PROGRAM IL
VAR
	RANGE_PG_PS1:RANGEJD;
	RANGE_PG_PS2:RANGEJD;
	RANGE_PG_PS3:RANGEJD;
	RANGE_PG_PS4:RANGEJD;
	RANGE_PG_PS5:RANGEJD;
	RANGE_PG_PS6:RANGEJD;
	RANGE_PG_PS7:RANGEJD;
	RANGE_PG_PS8:RANGEJD;
	RANGE_PG_PS9:RANGEJD;
	
	RANGE_MFC1:RANGEJD;
	RANGE_MFC2:RANGEJD;
	RANGE_MFC3:RANGEJD;
	RANGE_MFC4:RANGEJD;
	RANGE_MFC5:RANGEJD;
	RANGE_MFC6:RANGEJD;
	RANGE_MFC7:RANGEJD;
	RANGE_MFC8:RANGEJD;
	RANGE_MFC9:RANGEJD;
	
	RANGE_CHAMBER_HEATER1:RANGEJD;
	RANGE_CHAMBER_HEATER2:RANGEJD;
	RANGE_CHAMBER_HEATER3:RANGEJD;
	
	RANGE_LID_HEATER:RANGEJD;
	
	RANGE_STAGE_EDGE_HEATER:RANGEJD;
	RANGE_STAGE_CENTER_HEATER:RANGEJD;
	
	//INTERLOCK	
	TON_PrepareTransfer:TON;	
	TON_TransferWafer:TON;	
	TON_OpenGasValve:TON;	
	TON_CloseGasValve:TON;	
	TON_OpenCloseSlitValve:TON;
	
	ALWAYS_TRUE:BOOL:=TRUE;
END_VAR
VAR // added by the converter: edge detectors and wires of the graphical bodies
    _w1, _w2, _w3, _w4, _w5, _w6 : BOOL;
END_VAR

VALVE();
Temp();
SYS();
SPLC();
ACT_HEATER();
ACT_MFC();
ACT_MFC();

//TMP Pressure OUT OF RANGE
	IF GV.PMConfig.TurboN2Pressure	<=	GV.TurboN2PurgePressure
		THEN
		PM.INFO.Alarm.TurboN2PurgePressureOutOfRange:=TRUE;
		ELSE
		PM.INFO.Alarm.TurboN2PurgePressureOutOfRange:=FALSE;	
	END_IF
	
//PrepareTransfer TIMEOUT
	TON_PrepareTransfer(IN:= GV_IL.STATUS_PrepareTransfer, PT:=INT_TO_TIME(GV.PMConfig.PrepareTransferTimeout)*1000 , Q=> , ET=> );	
	IF TON_PrepareTransfer.Q
		THEN
		PM.INFO.Alarm.PrepareTransferTimerout:=TRUE;
		ELSE
		PM.INFO.Alarm.PrepareTransferTimerout:=FALSE;
	END_IF
	
//TransferWafer TIMEOUT
	TON_TransferWafer(IN:=GV_IL.STATUS_TransferWafer , PT:= INT_TO_TIME(GV.PMConfig.TransferWaferTimeout)*1000, Q=> , ET=> );
	IF TON_TransferWafer.Q
		THEN
		PM.INFO.Alarm.TransferWaferTimeout:=TRUE;
		ELSE
		PM.INFO.Alarm.TransferWaferTimeout:=FALSE;	
	END_IF
	
//OpenGasValve TIMEOUT
	TON_OpenGasValve(IN:=GV_IL.STATUS_OpenGasValve , PT:= INT_TO_TIME(GV.PMConfig.OpenGasValveTimeout)*1000, Q=> , ET=> );
	IF TON_OpenGasValve.Q
		THEN
		PM.INFO.Alarm.OpenGasValveTimeout:=TRUE;
		ELSE 
		PM.INFO.Alarm.OpenGasValveTimeout:=FALSE;
	END_IF
	
//CloseGasValve TIMEOUT
	TON_CloseGasValve(IN:=GV_IL.STATUS_CloseGasValve , PT:= INT_TO_TIME(GV.PMConfig.CloseGasValveTimeout)*1000, Q=> , ET=> );
	IF TON_CloseGasValve.Q
		THEN
		PM.INFO.Alarm.CloseGasValveTimeout:=TRUE;
		ELSE
		PM.INFO.Alarm.CloseGasValveTimeout:=FALSE;
	END_IF
	
//OpenCloseSlitValve TIMEOUT
	TON_OpenCloseSlitValve(IN:=GV_IL.STATUS_OpenCloseSlitValve , PT:= INT_TO_TIME(GV.PMConfig.OpenCloseSlitValveTimeout)*1000, Q=> , ET=> );
	IF TON_OpenCloseSlitValve.Q
		THEN
		PM.INFO.Alarm.OpenCloseSlitValveTimeout:=TRUE;
		ELSE
		PM.INFO.Alarm.OpenCloseSlitValveTimeout:=FALSE;	
	END_IF
	
	
//PRESSURE ALARM
	//PM.INFO.Alarm.PRESSURE:=
	
//ALARM OR WARNING OCCUR
	GV.ALARM_OCC:=NOT (
				 	//PM.INFO.Alarm.PRESSURE
					PM.INFO.Alarm.MFC1	
				AND PM.INFO.Alarm.MFC2	
				AND	PM.INFO.Alarm.MFC3
				AND PM.INFO.Alarm.MFC4	
				AND PM.INFO.Alarm.MFC5	
				AND PM.INFO.Alarm.MFC6
				AND PM.INFO.Alarm.MFC7	
				AND PM.INFO.Alarm.MFC8	
				AND PM.INFO.Alarm.MFC9
				AND PM.INFO.Alarm.WALL_TEMP	
				AND PM.INFO.Alarm.LID_TEMP	
				AND PM.INFO.Alarm.STAGE_EDGE_TEMP	
				AND PM.INFO.Alarm.STAGE_CENTER_TEMP
				AND PM.INFO.Alarm.Gas1FlowPressureOutOfRange
				AND PM.INFO.Alarm.Gas2FlowPressureOutOfRange
				AND PM.INFO.Alarm.Gas3FlowPressureOutOfRange
				//AND PM.INFO.Alarm.Gas4FlowPressureOutOfRange
				AND PM.INFO.Alarm.Gas5FlowPressureOutOfRange
				AND PM.INFO.Alarm.Gas6FlowPressureOutOfRange
				//AND PM.INFO.Alarm.TurboN2PurgePressureOutOfRange
				//AND PM.INFO.Alarm.PrepareTransferTimerout
				//AND PM.INFO.Alarm.TransferWaferTimeout
				//AND PM.INFO.Alarm.OpenGasValveTimeout
				//AND PM.INFO.Alarm.CloseGasValveTimeout
				//AND PM.INFO.Alarm.OpenCloseSlitValveTimeout
				//AND PM.INFO.Alarm.ATMCheckTimeout
				//AND PM.INFO.Alarm.DRY_PUMP
				//AND PM.INFO.Alarm.PENDULUM_VALVE
				//AND PM.INFO.Alarm.TURBO_PUMP
				AND PM.INFO.Alarm.CHILLER1
				AND PM.INFO.Alarm.CHILLER2
				AND (PM.INFO.Alarm.TOLERANCE_PRESSURE				
				AND PM.INFO.Alarm.TOLERANCE_MFC1
				AND PM.INFO.Alarm.TOLERANCE_MFC2
				AND PM.INFO.Alarm.TOLERANCE_MFC3
				AND PM.INFO.Alarm.TOLERANCE_MFC4
				AND PM.INFO.Alarm.TOLERANCE_MFC5
				AND PM.INFO.Alarm.TOLERANCE_MFC6
				AND PM.INFO.Alarm.TOLERANCE_MFC7
				AND PM.INFO.Alarm.TOLERANCE_MFC8
				AND PM.INFO.Alarm.TOLERANCE_MFC9
				AND PM.INFO.Alarm.TOLERANCE_WALL_TEMP
				AND PM.INFO.Alarm.TOLERANCE_LID_TEMP
				AND PM.INFO.Alarm.TOLERANCE_STAGE_EDGE_TEMP
				AND PM.INFO.Alarm.TOLERANCE_STAGE_CENTER_TEMP)
				);

	GV.WARNING_OCC:=NOT (
					//PM.INFO.Warning.PRESSURE					
					PM.INFO.Warning.MFC1
				AND PM.INFO.Warning.MFC2
				AND PM.INFO.Warning.MFC3
				AND PM.INFO.Warning.MFC4
				AND PM.INFO.Warning.MFC5
				AND PM.INFO.Warning.MFC6
				AND PM.INFO.Warning.MFC7
				AND PM.INFO.Warning.MFC8
				AND PM.INFO.Warning.MFC9
				AND PM.INFO.Warning.WALL_TEMP
				AND PM.INFO.Warning.LID_TEMP
				AND PM.INFO.Warning.STAGE_EDGE_TEMP
				AND PM.INFO.Warning.STAGE_CENTER_TEMP
				AND PM.INFO.Warning.Gas1FlowPressureOutOfRange
				AND PM.INFO.Warning.Gas2FlowPressureOutOfRange
				AND PM.INFO.Warning.Gas3FlowPressureOutOfRange
				//AND PM.INFO.Warning.Gas4FlowPressureOutOfRange
				AND PM.INFO.Warning.Gas5FlowPressureOutOfRange
				AND PM.INFO.Warning.Gas6FlowPressureOutOfRange
				//AND PM.INFO.Warning.OpenCloseSlitValveTimeout
				AND PM.INFO.Warning.CHILLER1
				AND PM.INFO.Warning.CHILLER2
				AND (PM.INFO.Warning.TOLERANCE_PRESSURE
				AND PM.INFO.Warning.TOLERANCE_MFC1
				AND PM.INFO.Warning.TOLERANCE_MFC2
				AND PM.INFO.Warning.TOLERANCE_MFC3
				AND PM.INFO.Warning.TOLERANCE_MFC4
				AND PM.INFO.Warning.TOLERANCE_MFC5
				AND PM.INFO.Warning.TOLERANCE_MFC6
				AND PM.INFO.Warning.TOLERANCE_MFC7
				AND PM.INFO.Warning.TOLERANCE_MFC8
				AND PM.INFO.Warning.TOLERANCE_MFC9
				AND PM.INFO.Warning.TOLERANCE_WALL_TEMP
				AND PM.INFO.Warning.TOLERANCE_LID_TEMP
				AND PM.INFO.Warning.TOLERANCE_STAGE_EDGE_TEMP
				AND PM.INFO.Warning.TOLERANCE_STAGE_CENTER_TEMP)
				);

ACTION ACT_HEATER:
//CHAMBER HEATER
	RANGE_CHAMBER_HEATER1(
	ENABLE:= GV.ChamberHeater.HeaterTolerance_Enable,
	SV:= REAL_TO_LREAL(GV.AO.Chamber_Temp1_SV),
	PV:= REAL_TO_LREAL( GV.AI.Chamber_Temp1), 
	RANGE_ALARM_H:= ANY_TO_REAL(GV.ChamberHeater.HeaterAlarmRange.SV), 
	RANGE_ALARM_L:= ANY_TO_LREAL(GV.ChamberHeater.HeaterAlarmRange.SV), 
	RANGE_WARNING_H:= ANY_TO_LREAL(GV.ChamberHeater.HeaterWarningRange.SV), 
	RANGE_WARNING_L:= ANY_TO_LREAL(GV.ChamberHeater.HeaterWarningRange.SV), 
	TIME_ALARM:= ANY_TO_LREAL(GV.ChamberHeater.HeaterAlarmTime.SV), 
	TIME_WARNING:= ANY_TO_LREAL(GV.ChamberHeater.HeaterWarningTime.SV), 
	ALARM=> , 
	WARNING=> );
	
	RANGE_CHAMBER_HEATER2(
	ENABLE:= GV.ChamberHeater.HeaterTolerance_Enable,
	SV:= REAL_TO_LREAL(GV.AO.Chamber_Temp2_SV),
	PV:= REAL_TO_LREAL( GV.AI.Chamber_Temp2), 
	RANGE_ALARM_H:= ANY_TO_LREAL(GV.ChamberHeater.HeaterAlarmRange.SV), 
	RANGE_ALARM_L:= ANY_TO_LREAL(GV.ChamberHeater.HeaterAlarmRange.SV), 
	RANGE_WARNING_H:= ANY_TO_LREAL(GV.ChamberHeater.HeaterWarningRange.SV), 
	RANGE_WARNING_L:= ANY_TO_LREAL(GV.ChamberHeater.HeaterWarningRange.SV), 
	TIME_ALARM:= ANY_TO_LREAL(GV.ChamberHeater.HeaterAlarmTime.SV), 
	TIME_WARNING:= ANY_TO_LREAL(GV.ChamberHeater.HeaterWarningTime.SV), 
	ALARM=> , 
	WARNING=> );
	
	RANGE_CHAMBER_HEATER3(
	ENABLE:= GV.ChamberHeater.HeaterTolerance_Enable,
	SV:= REAL_TO_LREAL(GV.AO.Chamber_Temp3_SV),
	PV:= REAL_TO_LREAL( GV.AI.Chamber_Temp3), 
	RANGE_ALARM_H:= ANY_TO_LREAL(GV.ChamberHeater.HeaterAlarmRange.SV), 
	RANGE_ALARM_L:= ANY_TO_LREAL(GV.ChamberHeater.HeaterAlarmRange.SV), 
	RANGE_WARNING_H:= ANY_TO_LREAL(GV.ChamberHeater.HeaterWarningRange.SV), 
	RANGE_WARNING_L:= ANY_TO_LREAL(GV.ChamberHeater.HeaterWarningRange.SV), 
	TIME_ALARM:= ANY_TO_LREAL(GV.ChamberHeater.HeaterAlarmTime.SV), 
	TIME_WARNING:= ANY_TO_LREAL(GV.ChamberHeater.HeaterWarningTime.SV), 
	ALARM=> , 
	WARNING=> );
	
	PM.INFO.Alarm.WALL_TEMP:=	RANGE_CHAMBER_HEATER1.ALARM 
							AND RANGE_CHAMBER_HEATER2.ALARM 
							AND RANGE_CHAMBER_HEATER3.ALARM
								;
	PM.INFO.Warning.WALL_TEMP:=	RANGE_CHAMBER_HEATER1.WARNING 
							AND RANGE_CHAMBER_HEATER2.WARNING 
							AND RANGE_CHAMBER_HEATER3.WARNING
								;
//LID HEATER
	RANGE_LID_HEATER(
	ENABLE:= GV.LidHeater.HeaterTolerance_Enable,
	SV:= REAL_TO_LREAL(GV.AO.LID_Temp_SV),
	PV:= REAL_TO_LREAL( GV.AI.Lid_Temp), 
	RANGE_ALARM_H:= ANY_TO_LREAL(GV.LidHeater.HeaterAlarmRange.SV), 
	RANGE_ALARM_L:= ANY_TO_LREAL(GV.LidHeater.HeaterAlarmRange.SV), 
	RANGE_WARNING_H:= ANY_TO_LREAL(GV.LidHeater.HeaterWarningRange.SV), 
	RANGE_WARNING_L:= ANY_TO_LREAL(GV.LidHeater.HeaterWarningRange.SV), 
	TIME_ALARM:= ANY_TO_LREAL(GV.LidHeater.HeaterAlarmTime.SV), 
	TIME_WARNING:= ANY_TO_LREAL(GV.LidHeater.HeaterWarningTime.SV), 
	ALARM=> , 
	WARNING=> );
	
	PM.INFO.Alarm.LID_TEMP	:=	RANGE_LID_HEATER.ALARM ;
	PM.INFO.Warning.LID_TEMP:=	RANGE_LID_HEATER.WARNING;
	
//STAGE HEATER
	RANGE_STAGE_CENTER_HEATER(
	ENABLE:= GV.Chiller.EnableAlarmTolerance,
	SV:= REAL_TO_LREAL(GV.AO.Chiller_Temp1_SV),
	PV:= REAL_TO_LREAL( GV.AI.CHILLER1_TEMP_PV), 
	RANGE_ALARM_H:= ANY_TO_LREAL(GV.Chiller.ToleranceAlarmRange.SV), 
	RANGE_ALARM_L:= ANY_TO_LREAL(GV.Chiller.ToleranceAlarmRange.SV), 
	RANGE_WARNING_H:= ANY_TO_LREAL(GV.Chiller.ToleranceAlarmRange.SV), 
	RANGE_WARNING_L:= ANY_TO_LREAL(GV.Chiller.ToleranceAlarmRange.SV), 
	TIME_ALARM:= ANY_TO_LREAL(GV.Chiller.ToleranceAlarmTime.SV), 
	TIME_WARNING:= ANY_TO_LREAL(GV.Chiller.ToleranceAlarmTime.SV), 
	ALARM=> , 
	WARNING=> );
	
	PM.INFO.Alarm.STAGE_CENTER_TEMP:=RANGE_STAGE_CENTER_HEATER.ALARM;
	PM.INFO.Warning.STAGE_CENTER_TEMP:=RANGE_STAGE_CENTER_HEATER.WARNING;
	PM.INFO.Alarm.CHILLER1:=NOT ECC.	CHILLER1_PV.Module2_Word[5].1;
	PM.INFO.Warning.CHILLER1:=NOT ECC.	CHILLER1_PV.Module2_Word[5].2;
	
	RANGE_STAGE_EDGE_HEATER(
	ENABLE:= GV.Chiller.EnableAlarmTolerance,
	SV:= REAL_TO_LREAL(GV.AO.Chiller_Temp2_SV),
	PV:= REAL_TO_LREAL( GV.AI.CHILLER2_TEMP_PV), 
	RANGE_ALARM_H:= ANY_TO_LREAL(GV.Chiller.ToleranceAlarmRange.SV), 
	RANGE_ALARM_L:= ANY_TO_LREAL(GV.Chiller.ToleranceAlarmRange.SV), 
	RANGE_WARNING_H:= ANY_TO_LREAL(GV.Chiller.ToleranceAlarmRange.SV), 
	RANGE_WARNING_L:= ANY_TO_LREAL(GV.Chiller.ToleranceAlarmRange.SV), 
	TIME_ALARM:= ANY_TO_LREAL(GV.Chiller.ToleranceAlarmTime.SV), 
	TIME_WARNING:= ANY_TO_LREAL(GV.Chiller.ToleranceAlarmTime.SV), 
	ALARM=> , 
	WARNING=> );
	
	PM.INFO.Alarm.STAGE_EDGE_TEMP:=RANGE_STAGE_EDGE_HEATER.ALARM;
	PM.INFO.Warning.STAGE_EDGE_TEMP:=RANGE_STAGE_EDGE_HEATER.WARNING;
	PM.INFO.Alarm.CHILLER2:=NOT ECC.	CHILLER2_PV.Module2_Word[5].1;
	PM.INFO.Warning.CHILLER2:=NOT ECC.	CHILLER2_PV.Module2_Word[5].2;
END_ACTION

ACTION ACT_MFC:
RANGE_MFC1(
	ENABLE:= GV.Mfcgas1.EnableAlarm AND GV.Mfcgas1.Enable,
	SV:= REAL_TO_LREAL(GV.AO.MFC1_Flow_Setpoint),
	PV:= REAL_TO_LREAL( GV.AI.MFC1_Flow), 
	RANGE_ALARM_H:= GV.Mfcgas1.AlarmRange.SV, 
	RANGE_ALARM_L:= GV.Mfcgas1.AlarmRange.SV, 
	RANGE_WARNING_H:= GV.Mfcgas1.WarningRange.SV, 
	RANGE_WARNING_L:= GV.Mfcgas1.WarningRange.SV, 
	TIME_ALARM:= GV.Mfcgas1.AlarmTime.SV, 
	TIME_WARNING:= GV.Mfcgas1.WarningTime.SV, 
	ALARM=> , 
	WARNING=> );
	
	RANGE_MFC2(
	ENABLE:= GV.Mfcgas2.EnableAlarm AND GV.Mfcgas2.Enable, 
	SV:= REAL_TO_LREAL(GV.AO.MFC2_Flow_Setpoint),
	PV:= REAL_TO_LREAL( GV.AI.MFC2_Flow), 
	RANGE_ALARM_H:= GV.Mfcgas2.AlarmRange.SV, 
	RANGE_ALARM_L:= GV.Mfcgas2.AlarmRange.SV, 
	RANGE_WARNING_H:= GV.Mfcgas2.WarningRange.SV, 
	RANGE_WARNING_L:= GV.Mfcgas2.WarningRange.SV, 
	TIME_ALARM:= GV.Mfcgas2.AlarmTime.SV, 
	TIME_WARNING:= GV.Mfcgas2.WarningTime.SV, 
	ALARM=> , 
	WARNING=> );

	RANGE_MFC3(	
	ENABLE:= GV.Mfcgas3.EnableAlarm AND GV.Mfcgas3.Enable, 
	SV:= REAL_TO_LREAL(GV.AO.MFC3_Flow_Setpoint),
	PV:= REAL_TO_LREAL( GV.AI.MFC3_Flow), 
	RANGE_ALARM_H:= GV.Mfcgas3.AlarmRange.SV, 
	RANGE_ALARM_L:= GV.Mfcgas3.AlarmRange.SV, 
	RANGE_WARNING_H:= GV.Mfcgas3.WarningRange.SV, 
	RANGE_WARNING_L:= GV.Mfcgas3.WarningRange.SV, 
	TIME_ALARM:= GV.Mfcgas3.AlarmTime.SV, 
	TIME_WARNING:= GV.Mfcgas3.WarningTime.SV,  
	ALARM=> , 
	WARNING=> );

	RANGE_MFC4(	
	ENABLE:= GV.Mfcgas4.EnableAlarm AND GV.Mfcgas4.Enable, 
	SV:= REAL_TO_LREAL(GV.AO.MFC4_Flow_Setpoint),
	PV:= REAL_TO_LREAL( GV.AI.MFC4_Flow), 
	RANGE_ALARM_H:= GV.Mfcgas4.AlarmRange.SV, 
	RANGE_ALARM_L:= GV.Mfcgas4.AlarmRange.SV, 
	RANGE_WARNING_H:= GV.Mfcgas4.WarningRange.SV, 
	RANGE_WARNING_L:= GV.Mfcgas4.WarningRange.SV, 
	TIME_ALARM:= GV.Mfcgas4.AlarmTime.SV, 
	TIME_WARNING:= GV.Mfcgas4.WarningTime.SV, 
	ALARM=> , 
	WARNING=> );
	
	RANGE_MFC5(	
	ENABLE:= GV.Mfcgas5.EnableAlarm AND GV.Mfcgas5.Enable, 
	SV:= REAL_TO_LREAL(GV.AO.MFC5_Flow_Setpoint),
	PV:= REAL_TO_LREAL( GV.AI.MFC5_Flow), 
	RANGE_ALARM_H:= GV.Mfcgas5.AlarmRange.SV, 
	RANGE_ALARM_L:= GV.Mfcgas5.AlarmRange.SV, 
	RANGE_WARNING_H:= GV.Mfcgas5.WarningRange.SV, 
	RANGE_WARNING_L:= GV.Mfcgas5.WarningRange.SV, 
	TIME_ALARM:= GV.Mfcgas5.AlarmTime.SV, 
	TIME_WARNING:= GV.Mfcgas5.WarningTime.SV, 
	ALARM=> , 
	WARNING=> );

	RANGE_MFC6(	
	ENABLE:= GV.Mfcgas6.EnableAlarm AND GV.Mfcgas6.Enable, 
	SV:= REAL_TO_LREAL(GV.AO.MFC6_Flow_Setpoint),
	PV:= REAL_TO_LREAL( GV.AI.MFC6_Flow), 
	RANGE_ALARM_H:= GV.Mfcgas6.AlarmRange.SV, 
	RANGE_ALARM_L:= GV.Mfcgas6.AlarmRange.SV, 
	RANGE_WARNING_H:= GV.Mfcgas6.WarningRange.SV, 
	RANGE_WARNING_L:= GV.Mfcgas6.WarningRange.SV, 
	TIME_ALARM:= GV.Mfcgas6.AlarmTime.SV, 
	TIME_WARNING:= GV.Mfcgas6.WarningTime.SV,  
	ALARM=> , 
	WARNING=> );

	RANGE_MFC7(	
	ENABLE:= GV.Mfcgas7.EnableAlarm AND GV.Mfcgas7.Enable, 
	SV:= REAL_TO_LREAL(GV.AO.MFC7_Flow_Setpoint),
	PV:= REAL_TO_LREAL( GV.AI.MFC7_Flow), 
	RANGE_ALARM_H:= GV.Mfcgas7.AlarmRange.SV, 
	RANGE_ALARM_L:= GV.Mfcgas7.AlarmRange.SV, 
	RANGE_WARNING_H:= GV.Mfcgas7.WarningRange.SV, 
	RANGE_WARNING_L:= GV.Mfcgas7.WarningRange.SV, 
	TIME_ALARM:= GV.Mfcgas7.AlarmTime.SV, 
	TIME_WARNING:= GV.Mfcgas7.WarningTime.SV, 
	ALARM=> , 
	WARNING=> );
(*
	RANGE_MFC8(	
	ENABLE:= GV.Mfcgas8.EnableAlarm AND GV.Mfcgas8.Enable, 
	PV:= REAL_TO_LREAL( GV.AI.MFC8_Flow), 
	RANGE_ALARM_H:= GV.Mfcgas8.AlarmRange.MaxSV, 
	RANGE_ALARM_L:= 0, 
	RANGE_WARNING_H:= GV.Mfcgas8.WarningRange.MaxSV, 
	RANGE_WARNING_L:= 0, 
	TIME_ALARM:= GV.Mfcgas8.AlarmTime.SV, 
	TIME_WARNING:= GV.Mfcgas8.WarningTime.SV, 
	ALARM=> , 
	WARNING=> );

	RANGE_MFC9(	
	ENABLE:= GV.Mfcgas9.EnableAlarm AND GV.Mfcgas9.Enable, 
	PV:= REAL_TO_LREAL( GV.AI.MFC9_Flow), 
	RANGE_ALARM_H:= GV.Mfcgas9.AlarmRange.MaxSV, 
	RANGE_ALARM_L:= 0, 
	RANGE_WARNING_H:= GV.Mfcgas9.WarningRange.MaxSV, 
	RANGE_WARNING_L:= 0, 
	TIME_ALARM:= GV.Mfcgas9.AlarmTime.SV, 
	TIME_WARNING:= GV.Mfcgas9.WarningTime.SV, 
	ALARM=> , 
	WARNING=> );
*)	
	
	PM.Info.Alarm.MFC1:=  RANGE_MFC1.ALARM;
	PM.INFO.Alarm.MFC2:=  RANGE_MFC2.ALARM;
	PM.INFO.Alarm.MFC3:=  RANGE_MFC3.ALARM;
	PM.INFO.Alarm.MFC4:=  RANGE_MFC4.ALARM;
	PM.INFO.Alarm.MFC5:=  RANGE_MFC5.ALARM;
	PM.INFO.Alarm.MFC6:=  RANGE_MFC6.ALARM;
	PM.INFO.Alarm.MFC7:=  RANGE_MFC7.ALARM;
	PM.INFO.Alarm.MFC8:=  RANGE_MFC8.ALARM OR TRUE;
	PM.INFO.Alarm.MFC9:=  RANGE_MFC9.ALARM OR TRUE;
	
	PM.INFO.warning.MFC1:=  RANGE_MFC1.warning;
	PM.INFO.warning.MFC2:=  RANGE_MFC2.warning;
	PM.INFO.warning.MFC3:=  RANGE_MFC3.warning;
	PM.INFO.warning.MFC4:=  RANGE_MFC4.warning;
	PM.INFO.warning.MFC5:=  RANGE_MFC5.warning;
	PM.INFO.warning.MFC6:=  RANGE_MFC6.warning;
	PM.INFO.warning.MFC7:=  RANGE_MFC7.warning;
	PM.INFO.warning.MFC8:=  RANGE_MFC8.warning OR TRUE;
	PM.INFO.warning.MFC9:=  RANGE_MFC9.warning OR TRUE;
END_ACTION

ACTION ACT_PG_PS:
RANGE_PG_PS1(
	ENABLE:=TRUE,
	SV:= 270,
	PV:= GV.AI.PG_PS1_VALUE, 
	RANGE_ALARM_H:= GV.PMConfig.GasFlowPressureAlarmRange, 
	RANGE_ALARM_L:= GV.PMConfig.GasFlowPressureAlarmRange, 
	RANGE_WARNING_H:= GV.PMConfig.GasFlowPressureWarningRange, 
	RANGE_WARNING_L:= GV.PMConfig.GasFlowPressureWarningRange, 
	TIME_ALARM:= GV.PMConfig.GasFlowPressureAlarmTime, 
	TIME_WARNING:= GV.PMConfig.GasFlowPressureWarningTime, 
	ALARM=> , 
	WARNING=> );
	
	RANGE_PG_PS2(
	ENABLE:=TRUE,
	SV:= 270 ,
	PV:= GV.AI.PG_PS2_VALUE, 
	RANGE_ALARM_H:= GV.PMConfig.GasFlowPressureAlarmRange, 
	RANGE_ALARM_L:= GV.PMConfig.GasFlowPressureAlarmRange, 
	RANGE_WARNING_H:= GV.PMConfig.GasFlowPressureWarningRange, 
	RANGE_WARNING_L:= GV.PMConfig.GasFlowPressureWarningRange, 
	TIME_ALARM:= GV.PMConfig.GasFlowPressureAlarmTime, 
	TIME_WARNING:= GV.PMConfig.GasFlowPressureWarningTime, 
	ALARM=> , 
	WARNING=> );
	
	RANGE_PG_PS3(
	ENABLE:=TRUE,
	SV:= 270 ,
	PV:= GV.AI.PG_PS3_VALUE, 
	RANGE_ALARM_H:= GV.PMConfig.GasFlowPressureAlarmRange, 
	RANGE_ALARM_L:= GV.PMConfig.GasFlowPressureAlarmRange, 
	RANGE_WARNING_H:= GV.PMConfig.GasFlowPressureWarningRange, 
	RANGE_WARNING_L:= GV.PMConfig.GasFlowPressureWarningRange, 
	TIME_ALARM:= GV.PMConfig.GasFlowPressureAlarmTime, 
	TIME_WARNING:= GV.PMConfig.GasFlowPressureWarningTime, 
	ALARM=> , 
	WARNING=> );
	
	RANGE_PG_PS4(
	ENABLE:=TRUE,
	SV:=25,
	PV:= GV.AI.PG_PS4_VALUE, 
	RANGE_ALARM_H:= GV.PMConfig.GasFlowPressureAlarmRange, 
	RANGE_ALARM_L:= GV.PMConfig.GasFlowPressureAlarmRange, 
	RANGE_WARNING_H:= GV.PMConfig.GasFlowPressureWarningRange, 
	RANGE_WARNING_L:= GV.PMConfig.GasFlowPressureWarningRange, 
	TIME_ALARM:= GV.PMConfig.GasFlowPressureAlarmTime, 
	TIME_WARNING:= GV.PMConfig.GasFlowPressureWarningTime, 
	ALARM=> , 
	WARNING=> );
	
	RANGE_PG_PS5(
	ENABLE:=TRUE,
	SV:= 270,
	PV:= GV.AI.PG_PS5_VALUE, 
	RANGE_ALARM_H:= GV.PMConfig.GasFlowPressureAlarmRange, 
	RANGE_ALARM_L:= GV.PMConfig.GasFlowPressureAlarmRange, 
	RANGE_WARNING_H:= GV.PMConfig.GasFlowPressureWarningRange, 
	RANGE_WARNING_L:= GV.PMConfig.GasFlowPressureWarningRange, 
	TIME_ALARM:= GV.PMConfig.GasFlowPressureAlarmTime, 
	TIME_WARNING:= GV.PMConfig.GasFlowPressureWarningTime, 
	ALARM=> , 
	WARNING=> );
	
	RANGE_PG_PS6(
	ENABLE:=TRUE,
	SV:=270,
	PV:= GV.AI.PG_PS6_VALUE, 
	RANGE_ALARM_H:= GV.PMConfig.GasFlowPressureAlarmRange, 
	RANGE_ALARM_L:= GV.PMConfig.GasFlowPressureAlarmRange, 
	RANGE_WARNING_H:= GV.PMConfig.GasFlowPressureWarningRange, 
	RANGE_WARNING_L:= GV.PMConfig.GasFlowPressureWarningRange, 
	TIME_ALARM:= GV.PMConfig.GasFlowPressureAlarmTime, 
	TIME_WARNING:= GV.PMConfig.GasFlowPressureWarningTime, 
	ALARM=> , 
	WARNING=> );
	
	RANGE_PG_PS7(
	ENABLE:=TRUE,
	PV:= GV.AI.PG_PS7_VALUE, 
	RANGE_ALARM_H:= GV.PMConfig.GasFlowPressureAlarmRange, 
	RANGE_ALARM_L:= GV.PMConfig.GasFlowPressureAlarmRange, 
	RANGE_WARNING_H:= GV.PMConfig.GasFlowPressureWarningRange, 
	RANGE_WARNING_L:= GV.PMConfig.GasFlowPressureWarningRange, 
	TIME_ALARM:= GV.PMConfig.GasFlowPressureAlarmTime, 
	TIME_WARNING:= GV.PMConfig.GasFlowPressureWarningTime, 
	ALARM=> , 
	WARNING=> );
	
	RANGE_PG_PS8(
	ENABLE:=TRUE,
	PV:= GV.AI.PG_PS8_VALUE, 
	RANGE_ALARM_H:= GV.PMConfig.GasFlowPressureAlarmRange, 
	RANGE_ALARM_L:= GV.PMConfig.GasFlowPressureAlarmRange, 
	RANGE_WARNING_H:= GV.PMConfig.GasFlowPressureWarningRange, 
	RANGE_WARNING_L:= GV.PMConfig.GasFlowPressureWarningRange, 
	TIME_ALARM:= GV.PMConfig.GasFlowPressureAlarmTime, 
	TIME_WARNING:= GV.PMConfig.GasFlowPressureWarningTime, 
	ALARM=> , 
	WARNING=> );
	
	RANGE_PG_PS9(
	ENABLE:=TRUE,
	PV:= GV.AI.PG_PS9_VALUE, 
	RANGE_ALARM_H:= GV.PMConfig.GasFlowPressureAlarmRange, 
	RANGE_ALARM_L:= GV.PMConfig.GasFlowPressureAlarmRange, 
	RANGE_WARNING_H:= GV.PMConfig.GasFlowPressureWarningRange, 
	RANGE_WARNING_L:= GV.PMConfig.GasFlowPressureWarningRange, 
	TIME_ALARM:= GV.PMConfig.GasFlowPressureAlarmTime, 
	TIME_WARNING:= GV.PMConfig.GasFlowPressureWarningTime, 
	ALARM=> , 
	WARNING=> );
	
	PM.INFO.Alarm.Gas1FlowPressureOutOfRange:=  RANGE_PG_PS1.ALARM;
	PM.INFO.Alarm.Gas2FlowPressureOutOfRange:=  RANGE_PG_PS2.ALARM;
	PM.INFO.Alarm.Gas3FlowPressureOutOfRange:=  RANGE_PG_PS3.ALARM;	
	PM.INFO.Alarm.Gas4FlowPressureOutOfRange:=  RANGE_PG_PS4.ALARM OR TRUE;
	PM.INFO.Alarm.Gas5FlowPressureOutOfRange:=  RANGE_PG_PS5.ALARM;
	PM.INFO.Alarm.Gas6FlowPressureOutOfRange:=  RANGE_PG_PS6.ALARM;
	//PM.INFO.Alarm.Gas7FlowPressureOutOfRange:=  RANGE_PG_PS7.ALARM;
	//PM.INFO.Alarm.Gas8FlowPressureOutOfRange:=  RANGE_PG_PS8.ALARM;
	//PM.INFO.Alarm.Gas9FlowPressureOutOfRange:=  RANGE_PG_PS9.ALARM;

	PM.INFO.warning.Gas1FlowPressureOutOfRange:=  RANGE_PG_PS1.warning;
	PM.INFO.warning.Gas2FlowPressureOutOfRange:=  RANGE_PG_PS2.warning;
	PM.INFO.warning.Gas3FlowPressureOutOfRange:=  RANGE_PG_PS3.warning;
	PM.INFO.warning.Gas4FlowPressureOutOfRange:=  RANGE_PG_PS4.warning;
	PM.INFO.warning.Gas5FlowPressureOutOfRange:=  RANGE_PG_PS5.warning;
	PM.INFO.warning.Gas6FlowPressureOutOfRange:=  RANGE_PG_PS6.warning;
	//PM.INFO.warning.Gas7FlowPressureOutOfRange:=  RANGE_PG_PS7.warning;
	//PM.INFO.warning.Gas8FlowPressureOutOfRange:=  RANGE_PG_PS8.warning;
	//PM.INFO.warning.Gas9FlowPressureOutOfRange:=  RANGE_PG_PS9.warning;
END_ACTION

ACTION SPLC:
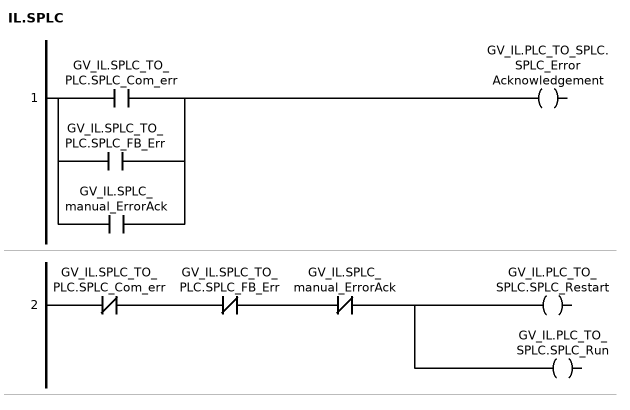
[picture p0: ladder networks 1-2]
// NETWORK 1
GV_IL.PLC_TO_SPLC.SPLC_ErrorAcknowledgement := GV_IL.SPLC_TO_PLC.SPLC_Com_err OR GV_IL.SPLC_TO_PLC.SPLC_FB_Err OR GV_IL.SPLC_manual_ErrorAck;

// NETWORK 2
_w1 := NOT GV_IL.SPLC_TO_PLC.SPLC_Com_err AND NOT GV_IL.SPLC_TO_PLC.SPLC_FB_Err AND NOT GV_IL.SPLC_manual_ErrorAck;
GV_IL.PLC_TO_SPLC.SPLC_Restart := _w1;
GV_IL.PLC_TO_SPLC.SPLC_Run := _w1;
END_ACTION

ACTION SYS:
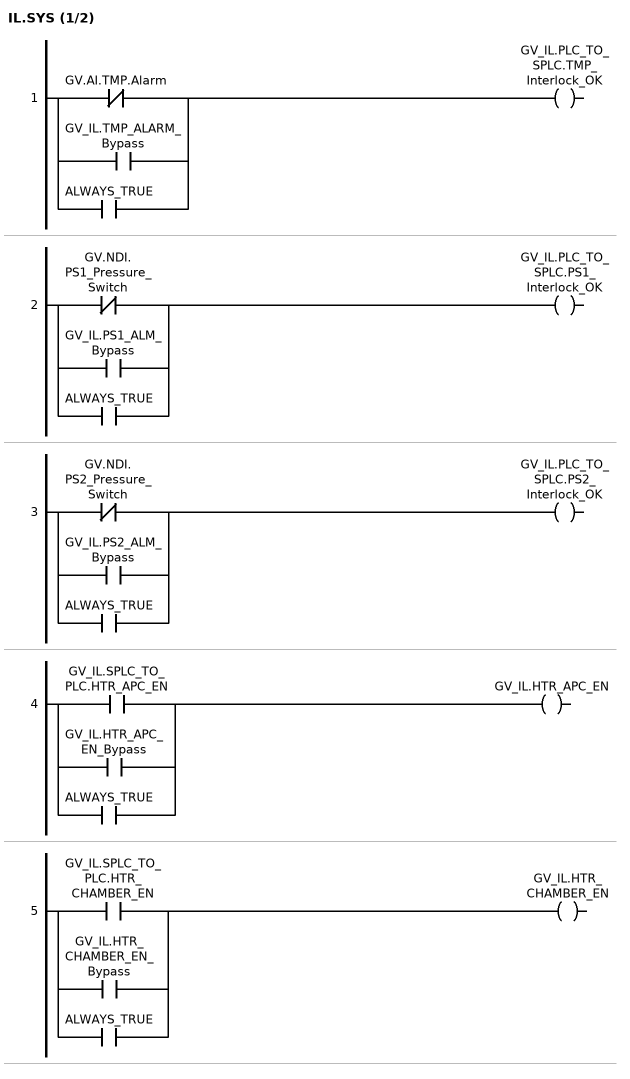
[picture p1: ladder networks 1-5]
// NETWORK 1
GV_IL.PLC_TO_SPLC.TMP_Interlock_OK := NOT GV.AI.TMP.Alarm OR GV_IL.TMP_ALARM_Bypass OR ALWAYS_TRUE;

// NETWORK 2
GV_IL.PLC_TO_SPLC.PS1_Interlock_OK := NOT (GV.NDI.	PS1_Pressure_Switch) OR GV_IL.PS1_ALM_Bypass OR ALWAYS_TRUE;

// NETWORK 3
GV_IL.PLC_TO_SPLC.PS2_Interlock_OK := NOT (GV.NDI.	PS2_Pressure_Switch) OR GV_IL.PS2_ALM_Bypass OR ALWAYS_TRUE;

// NETWORK 4
GV_IL.HTR_APC_EN := GV_IL.SPLC_TO_PLC.HTR_APC_EN OR GV_IL.HTR_APC_EN_Bypass OR ALWAYS_TRUE;

// NETWORK 5
GV_IL.HTR_CHAMBER_EN := GV_IL.SPLC_TO_PLC.HTR_CHAMBER_EN OR GV_IL.HTR_CHAMBER_EN_Bypass OR ALWAYS_TRUE;

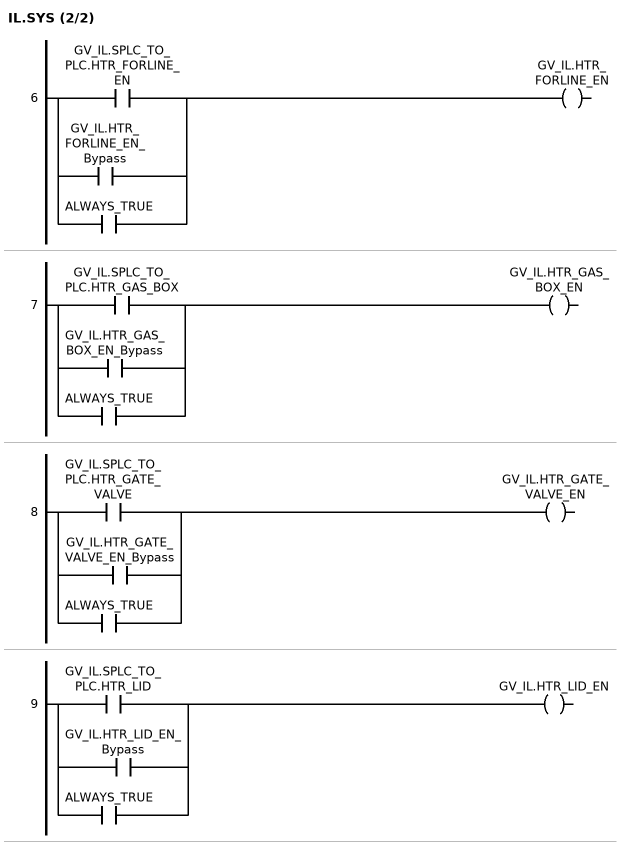
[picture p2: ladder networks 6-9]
// NETWORK 6
GV_IL.HTR_FORLINE_EN := GV_IL.SPLC_TO_PLC.HTR_FORLINE_EN OR GV_IL.HTR_FORLINE_EN_Bypass OR ALWAYS_TRUE;

// NETWORK 7
GV_IL.HTR_GAS_BOX_EN := GV_IL.SPLC_TO_PLC.HTR_GAS_BOX OR GV_IL.HTR_GAS_BOX_EN_Bypass OR ALWAYS_TRUE;

// NETWORK 8
GV_IL.HTR_GATE_VALVE_EN := GV_IL.SPLC_TO_PLC.HTR_GATE_VALVE OR GV_IL.HTR_GATE_VALVE_EN_Bypass OR ALWAYS_TRUE;

// NETWORK 9
GV_IL.HTR_LID_EN := GV_IL.SPLC_TO_PLC.HTR_LID OR GV_IL.HTR_LID_EN_Bypass OR ALWAYS_TRUE;
END_ACTION

ACTION Temp:
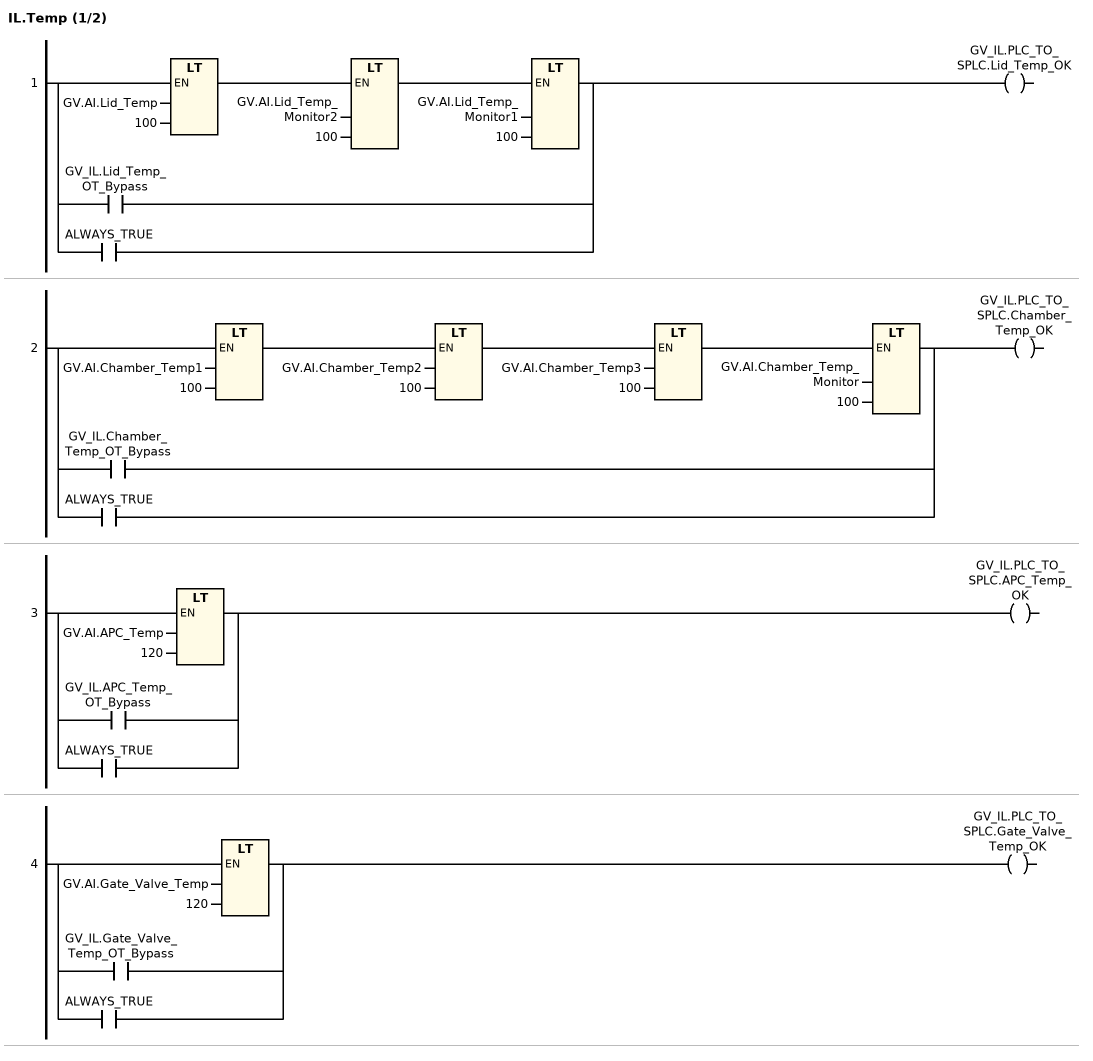
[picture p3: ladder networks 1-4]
// NETWORK 1
_w2 := GV_IL.Lid_Temp_OT_Bypass OR ALWAYS_TRUE;
IF NOT _w2 THEN
    _w2 := GV.AI.Lid_Temp < 100 AND GV.AI.Lid_Temp_Monitor2 < 100 AND GV.AI.Lid_Temp_Monitor1 < 100;
END_IF
GV_IL.PLC_TO_SPLC.Lid_Temp_OK := _w2;

// NETWORK 2
_w3 := GV_IL.Chamber_Temp_OT_Bypass OR ALWAYS_TRUE;
IF NOT _w3 THEN
    _w3 := GV.AI.Chamber_Temp1 < 100 AND GV.AI.Chamber_Temp2 < 100 AND GV.AI.Chamber_Temp3 < 100 AND GV.AI.Chamber_Temp_Monitor < 100;
END_IF
GV_IL.PLC_TO_SPLC.Chamber_Temp_OK := _w3;

// NETWORK 3
_w4 := GV_IL.APC_Temp_OT_Bypass OR ALWAYS_TRUE;
IF NOT _w4 THEN
    _w4 := GV.AI.APC_Temp < 120;
END_IF
GV_IL.PLC_TO_SPLC.APC_Temp_OK := _w4;

// NETWORK 4
_w5 := GV_IL.Gate_Valve_Temp_OT_Bypass OR ALWAYS_TRUE;
IF NOT _w5 THEN
    _w5 := GV.AI.Gate_Valve_Temp < 120;
END_IF
GV_IL.PLC_TO_SPLC.Gate_Valve_Temp_OK := _w5;

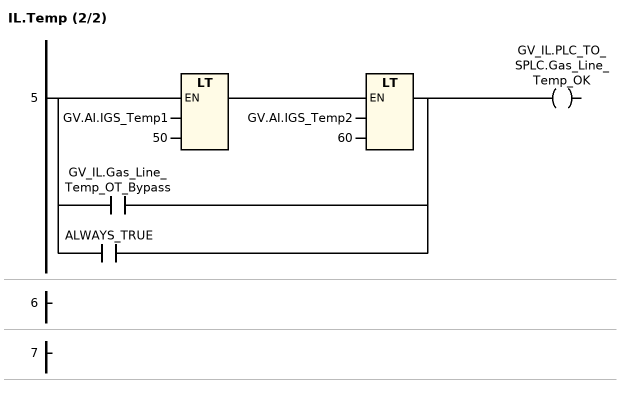
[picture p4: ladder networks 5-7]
// NETWORK 5
_w6 := GV_IL.Gas_Line_Temp_OT_Bypass OR ALWAYS_TRUE;
IF NOT _w6 THEN
    _w6 := GV.AI.IGS_Temp1 < 50 AND GV.AI.IGS_Temp2 < 60;
END_IF
GV_IL.PLC_TO_SPLC.Gas_Line_Temp_OK := _w6;

// NETWORK 6

// NETWORK 7
END_ACTION

ACTION VALVE:
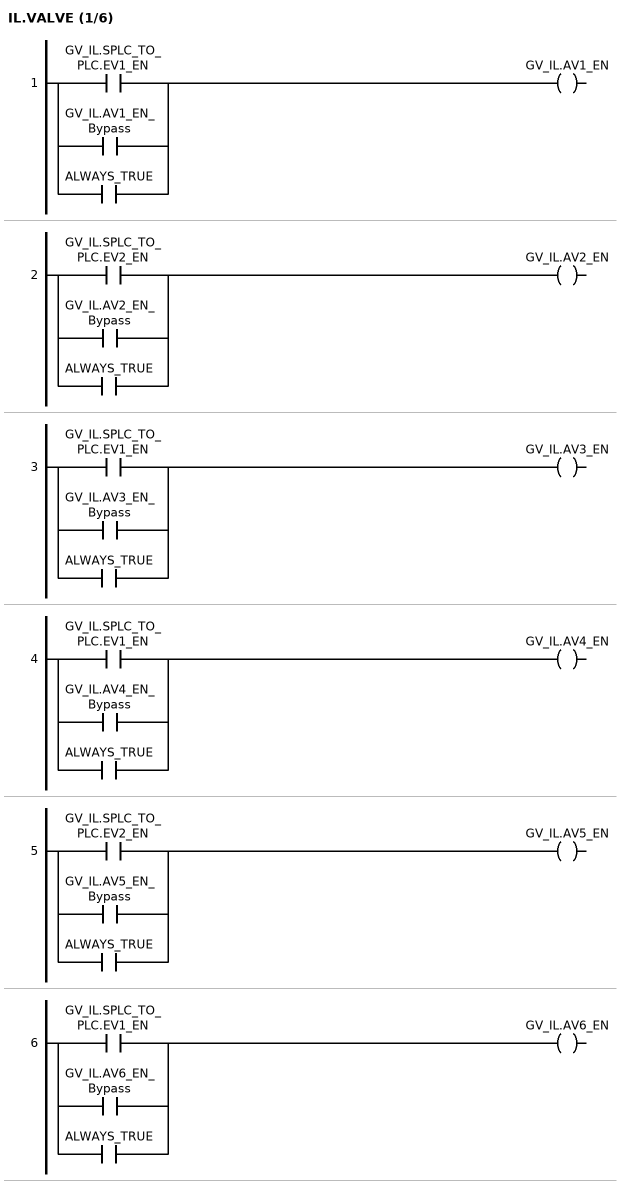
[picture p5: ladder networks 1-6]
// NETWORK 1
GV_IL.AV1_EN := GV_IL.SPLC_TO_PLC.EV1_EN OR GV_IL.AV1_EN_Bypass OR ALWAYS_TRUE;

// NETWORK 2
GV_IL.AV2_EN := GV_IL.SPLC_TO_PLC.EV2_EN OR GV_IL.AV2_EN_Bypass OR ALWAYS_TRUE;

// NETWORK 3
GV_IL.AV3_EN := GV_IL.SPLC_TO_PLC.EV1_EN OR GV_IL.AV3_EN_Bypass OR ALWAYS_TRUE;

// NETWORK 4
GV_IL.AV4_EN := GV_IL.SPLC_TO_PLC.EV1_EN OR GV_IL.AV4_EN_Bypass OR ALWAYS_TRUE;

// NETWORK 5
GV_IL.AV5_EN := GV_IL.SPLC_TO_PLC.EV2_EN OR GV_IL.AV5_EN_Bypass OR ALWAYS_TRUE;

// NETWORK 6
GV_IL.AV6_EN := GV_IL.SPLC_TO_PLC.EV1_EN OR GV_IL.AV6_EN_Bypass OR ALWAYS_TRUE;

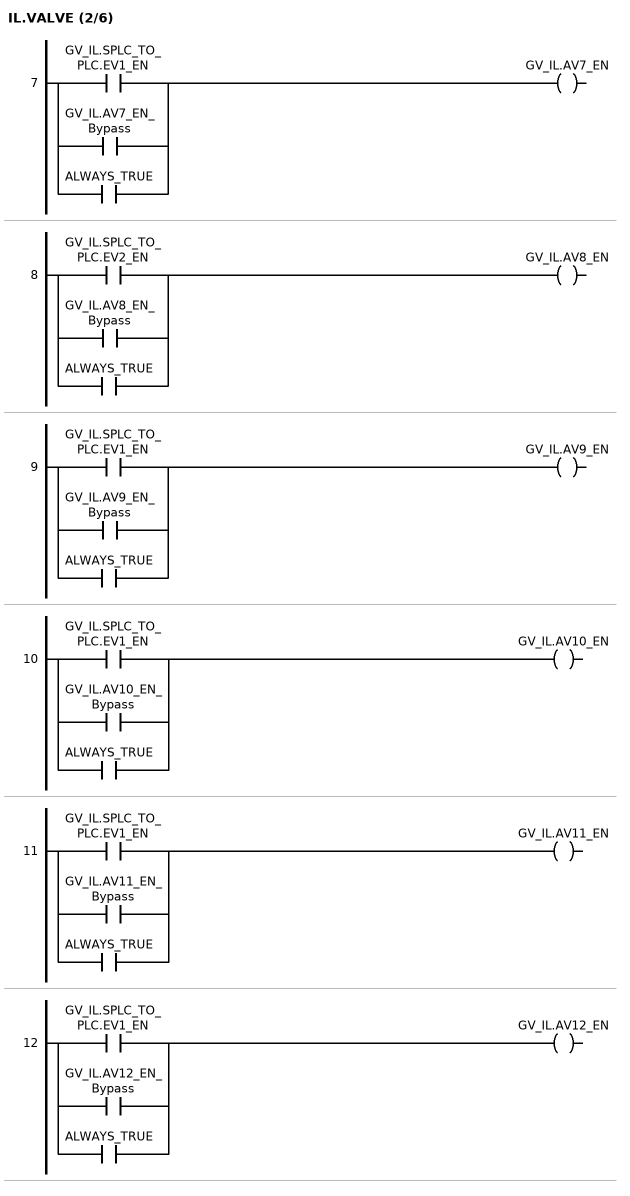
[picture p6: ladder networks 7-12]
// NETWORK 7
GV_IL.AV7_EN := GV_IL.SPLC_TO_PLC.EV1_EN OR GV_IL.AV7_EN_Bypass OR ALWAYS_TRUE;

// NETWORK 8
GV_IL.AV8_EN := GV_IL.SPLC_TO_PLC.EV2_EN OR GV_IL.AV8_EN_Bypass OR ALWAYS_TRUE;

// NETWORK 9
GV_IL.AV9_EN := GV_IL.SPLC_TO_PLC.EV1_EN OR GV_IL.AV9_EN_Bypass OR ALWAYS_TRUE;

// NETWORK 10
GV_IL.AV10_EN := GV_IL.SPLC_TO_PLC.EV1_EN OR GV_IL.AV10_EN_Bypass OR ALWAYS_TRUE;

// NETWORK 11
GV_IL.AV11_EN := GV_IL.SPLC_TO_PLC.EV1_EN OR GV_IL.AV11_EN_Bypass OR ALWAYS_TRUE;

// NETWORK 12
GV_IL.AV12_EN := GV_IL.SPLC_TO_PLC.EV1_EN OR GV_IL.AV12_EN_Bypass OR ALWAYS_TRUE;

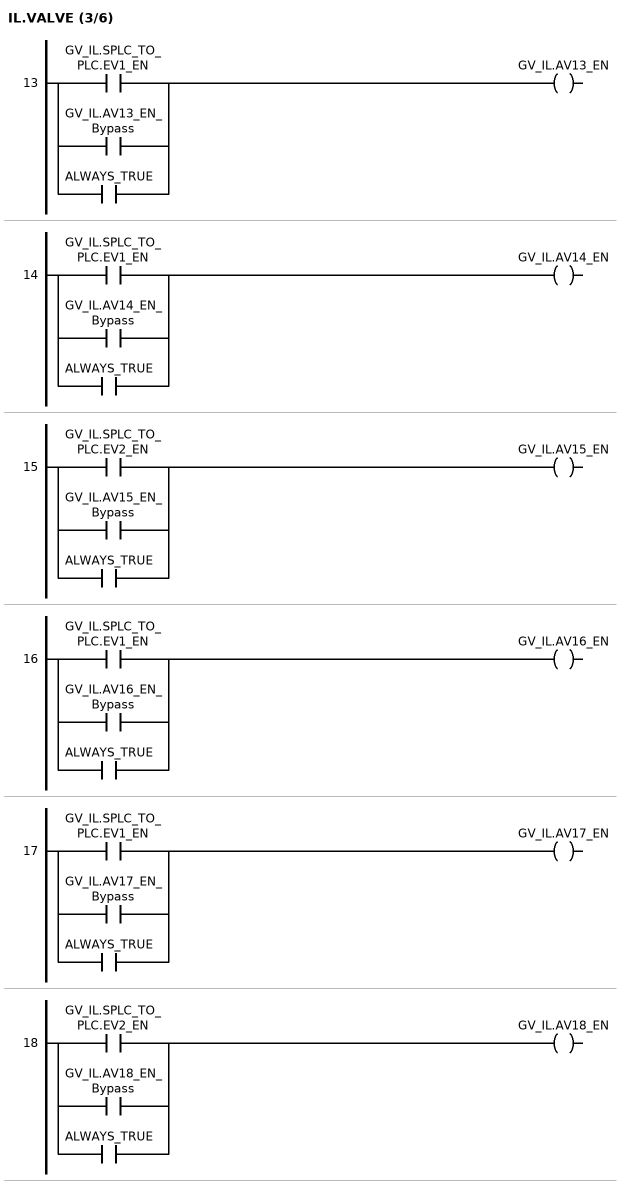
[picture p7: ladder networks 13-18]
// NETWORK 13
GV_IL.AV13_EN := GV_IL.SPLC_TO_PLC.EV1_EN OR GV_IL.AV13_EN_Bypass OR ALWAYS_TRUE;

// NETWORK 14
GV_IL.AV14_EN := GV_IL.SPLC_TO_PLC.EV1_EN OR GV_IL.AV14_EN_Bypass OR ALWAYS_TRUE;

// NETWORK 15
GV_IL.AV15_EN := GV_IL.SPLC_TO_PLC.EV2_EN OR GV_IL.AV15_EN_Bypass OR ALWAYS_TRUE;

// NETWORK 16
GV_IL.AV16_EN := GV_IL.SPLC_TO_PLC.EV1_EN OR GV_IL.AV16_EN_Bypass OR ALWAYS_TRUE;

// NETWORK 17
GV_IL.AV17_EN := GV_IL.SPLC_TO_PLC.EV1_EN OR GV_IL.AV17_EN_Bypass OR ALWAYS_TRUE;

// NETWORK 18
GV_IL.AV18_EN := GV_IL.SPLC_TO_PLC.EV2_EN OR GV_IL.AV18_EN_Bypass OR ALWAYS_TRUE;

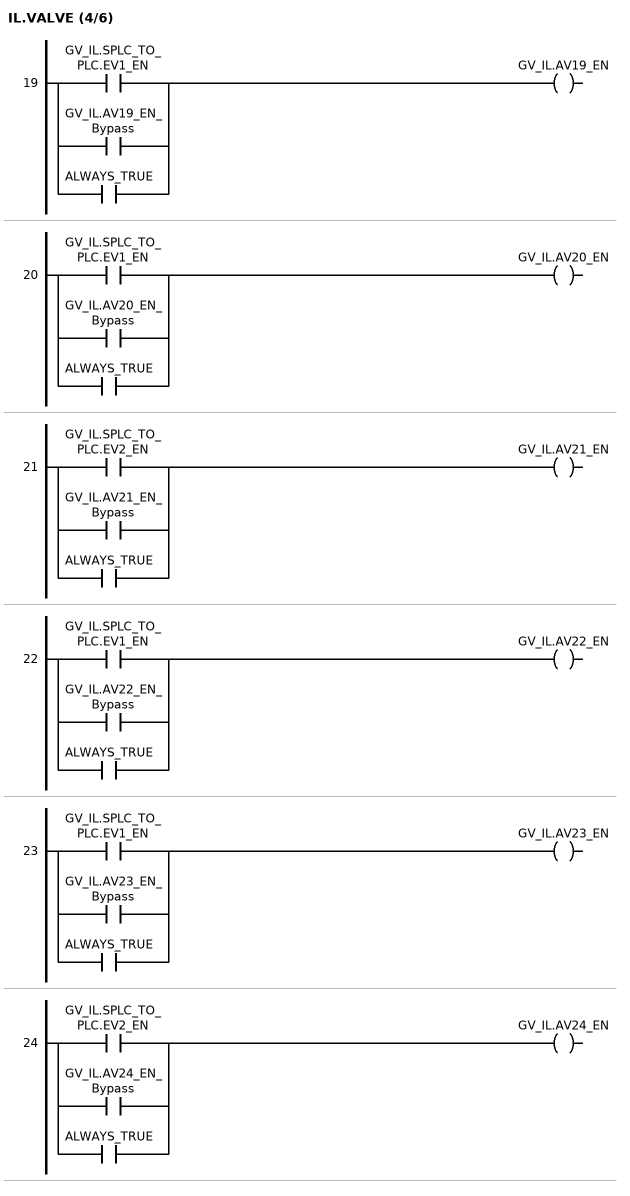
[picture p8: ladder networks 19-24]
// NETWORK 19
GV_IL.AV19_EN := GV_IL.SPLC_TO_PLC.EV1_EN OR GV_IL.AV19_EN_Bypass OR ALWAYS_TRUE;

// NETWORK 20
GV_IL.AV20_EN := GV_IL.SPLC_TO_PLC.EV1_EN OR GV_IL.AV20_EN_Bypass OR ALWAYS_TRUE;

// NETWORK 21
GV_IL.AV21_EN := GV_IL.SPLC_TO_PLC.EV2_EN OR GV_IL.AV21_EN_Bypass OR ALWAYS_TRUE;

// NETWORK 22
GV_IL.AV22_EN := GV_IL.SPLC_TO_PLC.EV1_EN OR GV_IL.AV22_EN_Bypass OR ALWAYS_TRUE;

// NETWORK 23
GV_IL.AV23_EN := GV_IL.SPLC_TO_PLC.EV1_EN OR GV_IL.AV23_EN_Bypass OR ALWAYS_TRUE;

// NETWORK 24
GV_IL.AV24_EN := GV_IL.SPLC_TO_PLC.EV2_EN OR GV_IL.AV24_EN_Bypass OR ALWAYS_TRUE;

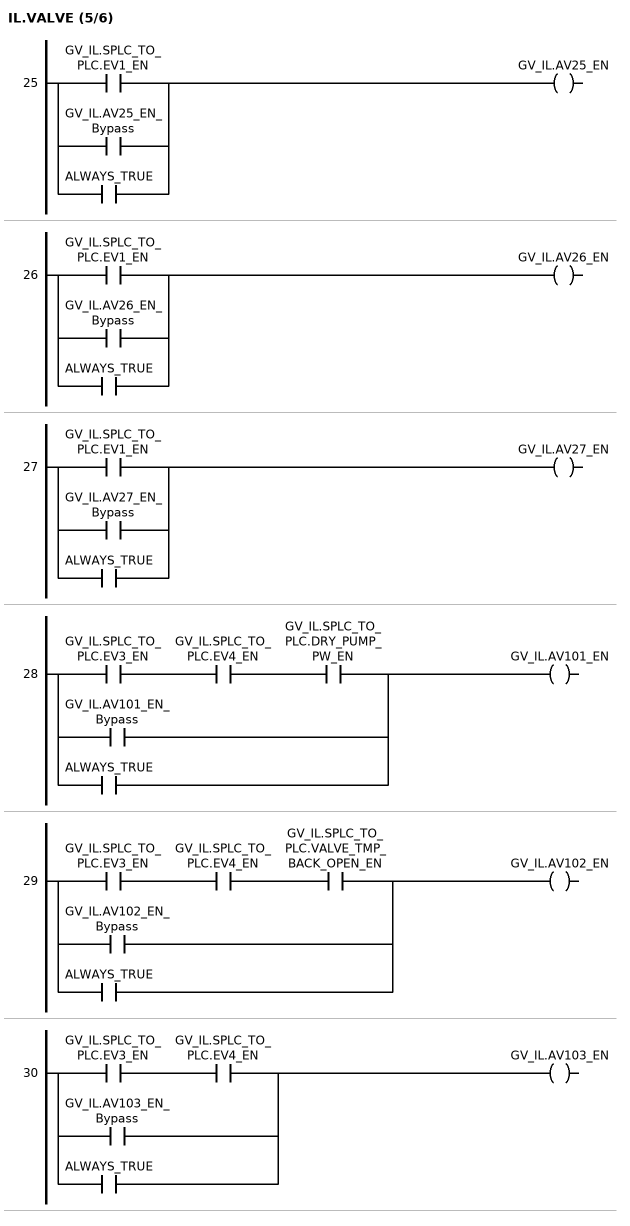
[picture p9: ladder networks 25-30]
// NETWORK 25
GV_IL.AV25_EN := GV_IL.SPLC_TO_PLC.EV1_EN OR GV_IL.AV25_EN_Bypass OR ALWAYS_TRUE;

// NETWORK 26
GV_IL.AV26_EN := GV_IL.SPLC_TO_PLC.EV1_EN OR GV_IL.AV26_EN_Bypass OR ALWAYS_TRUE;

// NETWORK 27
GV_IL.AV27_EN := GV_IL.SPLC_TO_PLC.EV1_EN OR GV_IL.AV27_EN_Bypass OR ALWAYS_TRUE;

// NETWORK 28
GV_IL.AV101_EN := GV_IL.SPLC_TO_PLC.EV3_EN AND GV_IL.SPLC_TO_PLC.EV4_EN AND GV_IL.SPLC_TO_PLC.DRY_PUMP_PW_EN OR GV_IL.AV101_EN_Bypass OR ALWAYS_TRUE;

// NETWORK 29
GV_IL.AV102_EN := GV_IL.SPLC_TO_PLC.EV3_EN AND GV_IL.SPLC_TO_PLC.EV4_EN AND GV_IL.SPLC_TO_PLC.VALVE_TMP_BACK_OPEN_EN OR GV_IL.AV102_EN_Bypass OR ALWAYS_TRUE;

// NETWORK 30
GV_IL.AV103_EN := GV_IL.SPLC_TO_PLC.EV3_EN AND GV_IL.SPLC_TO_PLC.EV4_EN OR GV_IL.AV103_EN_Bypass OR ALWAYS_TRUE;

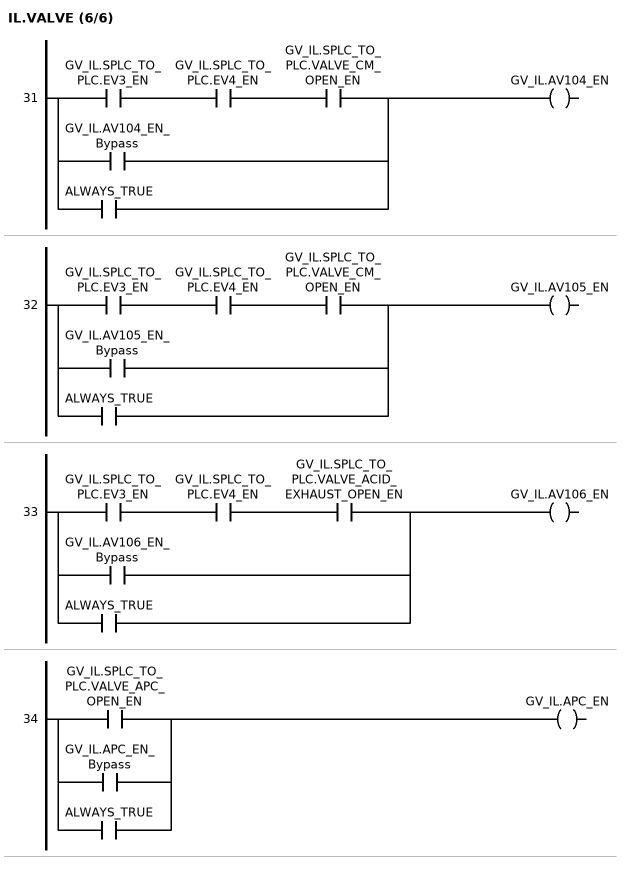
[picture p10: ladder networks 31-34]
// NETWORK 31
GV_IL.AV104_EN := GV_IL.SPLC_TO_PLC.EV3_EN AND GV_IL.SPLC_TO_PLC.EV4_EN AND GV_IL.SPLC_TO_PLC.VALVE_CM_OPEN_EN OR GV_IL.AV104_EN_Bypass OR ALWAYS_TRUE;

// NETWORK 32
GV_IL.AV105_EN := GV_IL.SPLC_TO_PLC.EV3_EN AND GV_IL.SPLC_TO_PLC.EV4_EN AND GV_IL.SPLC_TO_PLC.VALVE_CM_OPEN_EN OR GV_IL.AV105_EN_Bypass OR ALWAYS_TRUE;

// NETWORK 33
GV_IL.AV106_EN := GV_IL.SPLC_TO_PLC.EV3_EN AND GV_IL.SPLC_TO_PLC.EV4_EN AND GV_IL.SPLC_TO_PLC.VALVE_ACID_EXHAUST_OPEN_EN OR GV_IL.AV106_EN_Bypass OR ALWAYS_TRUE;

// NETWORK 34
GV_IL.APC_EN := GV_IL.SPLC_TO_PLC.VALVE_APC_OPEN_EN OR GV_IL.APC_EN_Bypass OR ALWAYS_TRUE;
END_ACTION

END_PROGRAM
